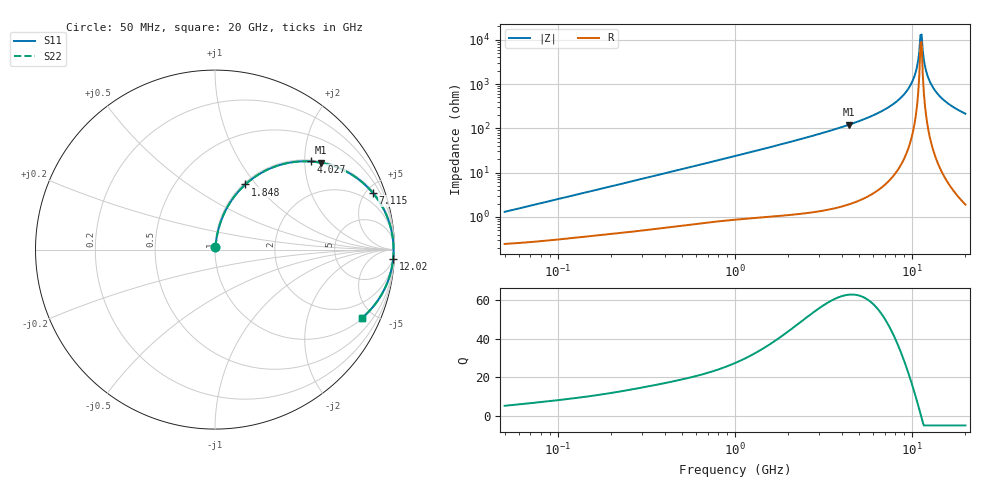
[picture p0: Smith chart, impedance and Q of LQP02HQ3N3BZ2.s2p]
!Murata Part Number: LQP02HQ3N3BZ2
!These Parameters are Measured in Series Mode Connection
!  o--[Z]--o
!Port1  Port2
!  o-------o
!Freq. Start=50[MHz] Stop=20[GHz], 401[Steps]
# Hz S RI R 50
!Freq.(Hz) S11(Real) S11(Imag) S21(Real) S21(Imag) S12(Real) S12(Imag) S22(Real) S22(Imag)
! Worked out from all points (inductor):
!   401 points, 50 MHz to 20 GHz, reference 50 ohm
!   read as one part in series: L = 4.04 nH near 51.52 MHz
!   highest Q = 62.8 at 4.406 GHz (marker M1), where L = 4.36 nH
!   self-resonance near 11.15 GHz
!   S11 on the Smith chart (normalised r, x): 50 MHz: 1.00, +0.03; 1.848 GHz: 1.02, +0.88; 4.027 GHz: 1.03, +2.14; 7.115 GHz: 1.11, +5.50; 12.02 GHz: 5, -38; 20 GHz: 1.04, -4.28
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5e7  0.00261 0.0127  0.9974 -0.0127  0.9974 -0.0127  0.00261 0.0127
1.364002e8  0.00463 0.0335  0.9954 -0.0335  0.9954 -0.0335  0.00463 0.0335
3.721004e8  0.0133 0.0878  0.9867 -0.0878  0.9867 -0.0878  0.0133 0.0878
1e9  0.0602 0.2203  0.9398 -0.2203  0.9398 -0.2203  0.0602 0.2203
1.848039e9  0.1694 0.3633  0.8306 -0.3633  0.8306 -0.3633  0.1694 0.3633
2.728004e9  0.3151 0.4552  0.6849 -0.4552  0.6849 -0.4552  0.3151 0.4552
4.026975e9  0.534 0.4909  0.466 -0.4909  0.466 -0.4909  0.534 0.4909
4.405649e9  0.5916 0.4836  0.4084 -0.4836  0.4084 -0.4836  0.5916 0.4836
7.114996e9  0.8784 0.3168  0.1216 -0.3168  0.1216 -0.3168  0.8784 0.3168
7.442007e9  0.8991 0.2906  0.1009 -0.2906  0.1009 -0.2906  0.8991 0.2906
8.774992e9  0.959 0.1829  0.041 -0.1829  0.041 -0.1829  0.959 0.1829
9.892087e9  0.985 0.0962  0.015 -0.0962  0.015 -0.0962  0.985 0.0962
1.050288e10  0.992 0.0513  0.008 -0.0513  0.008 -0.0513  0.992 0.0513
1.098561e10  0.9945 0.0172  0.00551 -0.0172  0.00551 -0.0172  0.9945 0.0172
1.115139e10  0.9948 0.00583  0.0052 -0.00583  0.0052 -0.00583  0.9948 0.00583
1.131968e10  0.9948 -0.00556  0.00515 0.00556  0.00515 0.00556  0.9948 -0.00556
1.149051e10  0.9946 -0.0169  0.00537 0.0169  0.00537 0.0169  0.9946 -0.0169
1.201863e10  0.9924 -0.051  0.00758 0.051  0.00758 0.051  0.9924 -0.051
1.276073e10  0.9858 -0.0961  0.0142 0.0961  0.0142 0.0961  0.9858 -0.0961
1.417136e10  0.9645 -0.1726  0.0355 0.1726  0.0355 0.1726  0.9645 -0.1726
1.646126e10  0.9139 -0.2734  0.0861 0.2734  0.0861 0.2734  0.9139 -0.2734
2e10  0.8183 -0.3812  0.1817 0.3812  0.1817 0.3812  0.8183 -0.3812
